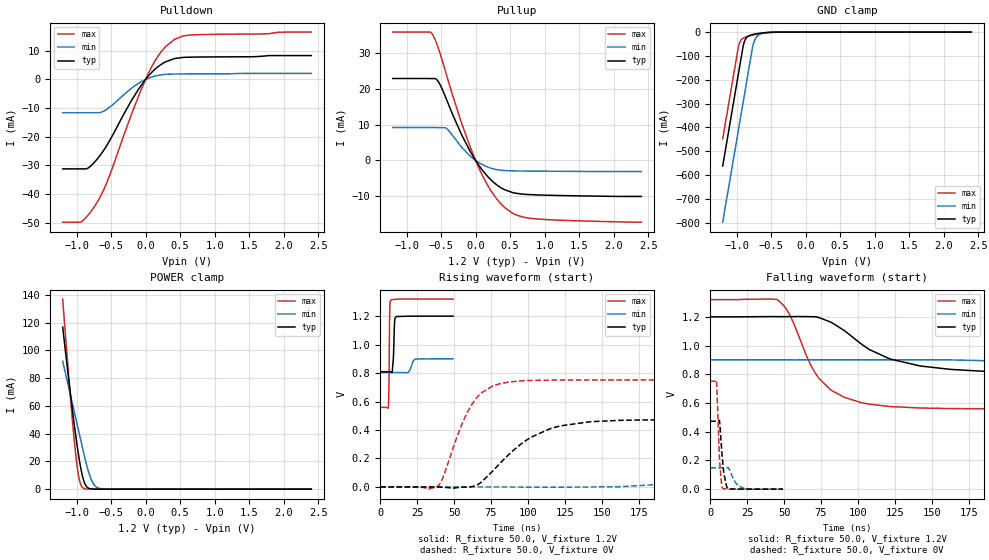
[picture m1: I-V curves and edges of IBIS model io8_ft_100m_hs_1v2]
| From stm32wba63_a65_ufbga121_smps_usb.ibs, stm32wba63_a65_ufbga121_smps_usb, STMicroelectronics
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[Model]   io8_ft_100m_hs_1v2
Model_type I/O
Polarity   Non-Inverting
Enable   Active-Low
| CAP_THRESHOLD on pad IOFT is "UDTCAPC" :
| Rising=30.0% of vddiom   Falling=70.0% of vddiom
| C_comp min and max val. don't necessarily correlate with the min and max pvt
| but are the smallest and greatest pad capacitance found.
| var   typ   min   max
C_comp   2.87220pF  2.79491pF  2.97971pF
|C_comp_pullup   1.64345pF  1.48389pF  1.78485pF
|C_comp_pulldown   1.22875pF  1.31102pF  1.19486pF
Vinl = 450.0mV
Vinh = 660.0mV
Vmeas = 600.0mV   | Reference voltage for timing measurements
Cref  = 50.0pF   | Timing specification test load capacitance value
Rref  = 1.0MOhm   | Timing specification test load resistance value
Vref  = 660.0mV   | Timing specification test load voltage
[Model Spec]
| TIME_THRESHOLD on pin ZIV11 is "CMOS" :
| Rising=50.0% of vdd   Falling=50.0% of vdd
Vinl 441.50000mV 335.50000mV 487.50000mV
Vinh 755.50000mV 552.50000mV 839.50000mV
| variable   typ   min   max
[Temperature Range] 25.0 140.0 -40.0
| variable   typ   min   max
[Voltage Range] 1.2V 900.0mV 1.32V
| variable   typ   min   max
[POWER Clamp Reference] 1.2V 900.0mV 1.32V
| variable   typ   min   max
[GND Clamp Reference] 0V 0V 0V
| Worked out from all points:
|   slope of the pulldown table from 0 to 0.18 V, typ, clamps not added: 40.6 ohm
|   slope of the pullup table from 0 to 0.18 V, typ, clamps not added: 39.4 ohm
|   GND clamp passes 1 mA (typ) near -0.51 V on its own axis
|   POWER clamp passes 1 mA (typ) near -0.83 V on its own axis
|   rising waveform, R_fixture 50.0, V_fixture 1.2V: 20-80 % time 787ps typ, 2.02ns min, 413ps max; typ from 0.809 V to 1.2 V
|   falling waveform, R_fixture 50.0, V_fixture 1.2V: 20-80 % time 41.7ns typ, 93.6ns min, 23.7ns max; typ from 1.2 V to 0.809 V
|   rising waveform, R_fixture 50.0, V_fixture 0V: 20-80 % time 33.9ns typ, 84.5ns min, 18.2ns max; typ from 0 V to 0.473 V
|   falling waveform, R_fixture 50.0, V_fixture 0V: 20-80 % time 2.55ns typ, 4.8ns min, 1.84ns max; typ from 0.473 V to 0 V
[POWER Clamp]
-1.2V     116.7mA    92.13mA    136.9mA
-1.09V    69.42mA    68.21mA    67.14mA
-1.02V    41.75mA    52.99mA    28.91mA
-990mV    30.98mA    46.47mA    16.09mA
-970mV    24.36mA    42.12mA    9.575mA
-940mV    15.59mA    35.6mA     3.485mA
-910mV    8.693mA    29.07mA    1.01mA
-860mV    2.259mA    18.59mA    104.6uA
-780mV    143.1uA    6.246mA    2.555uA
-720mV    16.22uA    1.846mA    157.1nA
-650mV    1.267uA    330.3uA    6.118nA
2.4V      0A         0A         0A
[GND Clamp]
-1.2V     -561.6mA   -797.4mA   -447.4mA
-980mV    -187.6mA   -423.4mA   -73.43mA
-960mV    -153.6mA   -389.4mA   -48.26mA
-900mV    -54.17mA   -287.4mA   -24.97mA
-870mV    -29.55mA   -236.4mA   -21.19mA
-830mV    -17.05mA   -168.4mA   -17.42mA
-760mV    -9.921mA   -54.55mA   -11.89mA
-730mV    -8.191mA   -29.78mA   -9.811mA
-690mV    -6.26mA    -14.49mA   -7.318mA
-600mV    -2.976mA   -4.315mA   -3.058mA
-380mV    -57.63uA   -251uA     -19.49uA
2.4V      872.8pA    204.8nA    349.4pA
| variable   typ   min   max
[Pullup Reference] 1.2V 900.0mV 1.32V
| variable   typ   min   max
[Pulldown Reference] 0V 0V 0V
[Pullup]
-1.2V     22.83mA    9.172mA    35.76mA
-660mV    22.81mA    9.172mA    35.76mA
-620mV    22.81mA    9.172mA    35mA
-540mV    21.98mA    9.133mA    31.33mA
-420mV    16.95mA    8.88mA     23.76mA
-200mV    7.069mA    3.642mA    10.26mA
0V        545.3fA    208.5pA    3fA
210mV     -5.173mA   -2.076mA   -8.052mA
420mV     -8.158mA   -2.82mA    -13.11mA
570mV     -9.105mA   -2.921mA   -15.05mA
790mV     -9.528mA   -2.972mA   -16.12mA
2.4V      -10.04mA   -3.075mA   -17.21mA
[Pulldown]
-1.2V     -31.2mA    -11.62mA   -49.78mA
-930mV    -31.2mA    -11.62mA   -49.64mA
-830mV    -30.86mA   -11.62mA   -47.25mA
-710mV    -28.04mA   -11.62mA   -43.19mA
-550mV    -22.55mA   -10.2mA    -35.3mA
-200mV    -7.146mA   -2.964mA   -11.89mA
40mV      1.171mA    405.8uA    2.092mA
130mV     3.416mA    1.118mA    6.182mA
230mV     5.302mA    1.613mA    9.763mA
420mV     7.288mA    1.898mA    13.99mA
670mV     7.779mA    1.924mA    15.51mA
2.4V      8.312mA    2.101mA    16.51mA
[Ramp]
dV/dt_r 283.7954mV/6.61137ns 88.9348mV/16.82284ns 450.99316mV/3.62072ns
dV/dt_f 234.65976mV/7.9358ns 57.89637mV/18.64358ns 456.73591mV/4.66138ns
R_load = 50.0
| Removed startup time: 0s 0s 0s  .
| Removed end time: 49.25ns.
[Rising Waveform]
R_fixture   = 50.0
V_fixture   = 1.2V
V_fixture_min = 900.0mV
V_fixture_max = 1.32V
0s        808.9mV    803.5mV    558.8mV
5.45ns    808.9mV    803.5mV    560mV
5.9ns     808.9mV    803.5mV    723.2mV
6.4ns     809mV      803.5mV    1.238V
7.05ns    808.5mV    803.5mV    1.312V
8.05ns    805.3mV    803.5mV    1.316V
8.85ns    900.4mV    803.5mV    1.316V
9.75ns    1.167V     803.5mV    1.318V
11.05ns   1.197V     803.5mV    1.319V
49.25ns   1.2V       899.8mV    1.32V
| Removed startup time: 0s 0s 0s  .
| Removed end time: 996.25ns.
[Falling Waveform]
R_fixture   = 50.0
V_fixture   = 1.2V
V_fixture_min = 900.0mV
V_fixture_max = 1.32V
0s        1.2V       900mV      1.32V
45.5ns    1.201V     900mV      1.318V
54.25ns   1.202V     900mV      1.204V
69.5ns    1.201V     900.6mV    836.3mV
81.25ns   1.165V     900.7mV    694.2mV
122ns     905.7mV    900.5mV    575.2mV
162.7ns   834mV      900.1mV    561.3mV
223.8ns   812.6mV    867.8mV    558.9mV
386.5ns   808.9mV    809.1mV    558.8mV
996.2ns   808.9mV    803.5mV    558.8mV
| Removed startup time: 0s 0s 0s  .
| Removed end time: 996.0ns.
[Rising Waveform]
R_fixture   = 50.0
V_fixture   = 0V
V_fixture_min = 0V
V_fixture_max = 0V
0s        4.648nV    215.3nV    3.229nV
39ns      -307.1uV   954.5nV    7.174mV
56.75ns   -980.7uV   387.7nV    474.5mV
65ns      11.28mV    -257.7nV   622.4mV
76.25ns   113mV      9.729uV    710.2mV
94.5ns    295.6mV    -628.2uV   744.4mV
122ns     429.3mV    -1.116mV   750.9mV
162.7ns   468.1mV    1.935mV    751.5mV
345.8ns   472.9mV    141mV      751.6mV
996ns     473mV      148.2mV    751.7mV
| Removed startup time: 0s 0s 0s  .
| Removed end time: 49.25ns.
[Falling Waveform]
R_fixture   = 50.0
V_fixture   = 0V
V_fixture_min = 0V
V_fixture_max = 0V
0s        473mV      148.3mV    751.7mV
4.2ns     473mV      148.3mV    753.9mV
6.25ns    474.3mV    148.3mV    215.8mV
7.4ns     319.5mV    148.3mV    59.94mV
8.15ns    217.7mV    148.3mV    8.874mV
9.1ns     118.6mV    148.3mV    3.153mV
12.05ns   3.482mV    151.4mV    808.1uV
17.1ns    778.8uV    45.68mV    183.8uV
22.15ns   277.1uV    8.183mV    54.27uV
49.25ns   3.151uV    119.5uV    50.81nV
